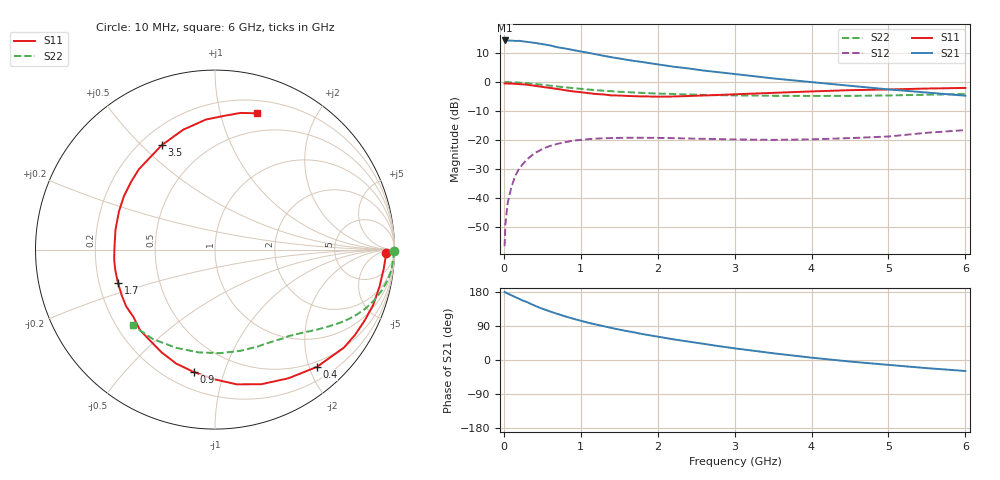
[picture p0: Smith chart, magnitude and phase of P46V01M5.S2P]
! SIEMENS Small Signal Semiconductors
! BFP182
! Si NPN RF Bipolar Junction Transistor in SOT143
! VCE = 6 V  IC = 1.5 mA
! Common Emitter S-Parameters:  March  1996
# GHz  S  MA  R  50
!  f  S11  S21  S12  S22
! GHz  MAG  ANG  MAG  ANG  MAG  ANG  MAG  ANG
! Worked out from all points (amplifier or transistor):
!   36 points, 10 MHz to 6 GHz, reference 50 ohm
!   highest |S21| = 14.3 dB at 10 MHz (marker M1)
!   |S21| within 3 dB of that: start of sweep to 844.1 MHz
!   unconditionally stable (mu >= 1): 2.442 GHz to end of sweep
!   at 250 MHz: K = 0.11, MSG = 21.1 dB, |S12| = -28.1 dB
!   at 1.4 GHz: K = 0.61, MSG = 13.9 dB, |S12| = -19.3 dB
!   at 6 GHz: K = 1.03, MAG = 4.9 dB, |S12| = -16.5 dB
!   S11 on the Smith chart (normalised r, x): 10 MHz: 35, -12; 400 MHz: 0.41, -2.13; 900 MHz: 0.30, -0.79; 1.7 GHz: 0.28, -0.15; 3.5 GHz: 0.28, +0.58; 6 GHz: 0.32, +1.30
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0.01  0.9503 -1.0  5.207 179.4  0.0015 84.5  0.9971 -0.4
0.02  0.9512 -2.6  5.205 178.7  0.0035 81.5  0.9995 -1.0
0.05  0.9462 -6.4  5.203 175.3  0.0084 88.0  0.9951 -2.4
0.1  0.9396 -12.6  5.177 170.7  0.0159 80.5  0.9915 -4.8
0.2  0.923 -25.2  5.125 161.2  0.0326 74.9  0.9786 -9.5
0.25  0.9136 -31.3  5.026 156.6  0.0393 71.3  0.9675 -11.8
0.4  0.8658 -49.0  4.735 143.5  0.0597 60.9  0.9295 -17.8
0.5  0.8254 -60.3  4.508 135.3  0.0703 54.6  0.8997 -21.5
0.6  0.7932 -71.0  4.278 128.2  0.0798 49.2  0.8686 -24.7
0.7  0.7604 -80.8  3.968 121.5  0.0868 44.4  0.8397 -27.4
0.8  0.7228 -90.2  3.783 115.0  0.0926 39.9  0.8123 -29.9
0.9  0.692 -99.9  3.567 109.1  0.0982 35.9  0.7876 -32.0
1.1  0.6454 -117.4  3.19 98.2  0.1043 29.1  0.7437 -35.9
1.4  0.5897 -140.3  2.675 84.6  0.1088 20.9  0.6965 -40.8
1.7  0.5715 -161.0  2.306 72.6  0.1102 15.6  0.6611 -45.1
1.9  0.5648 -174.0  2.113 65.1  0.1098 12.9  0.6429 -48.0
2.2  0.5652 168.9  1.844 54.7  0.1085 9.9  0.6243 -52.3
2.8  0.6015 140.8  1.476 36.4  0.1042 7.4  0.594 -62.2
3.5  0.6529 117.1  1.157 17.8  0.1014 8.3  0.5815 -75.8
4.5  0.726 94.1  0.864 -4.1  0.1086 13.7  0.58 -99.3
5.5  0.7747 79.4  0.661 -21.5  0.1343 17.6  0.6067 -124.7
6  0.7941 73.0  0.583 -29.0  0.1493 15.3  0.6241 -137.4
